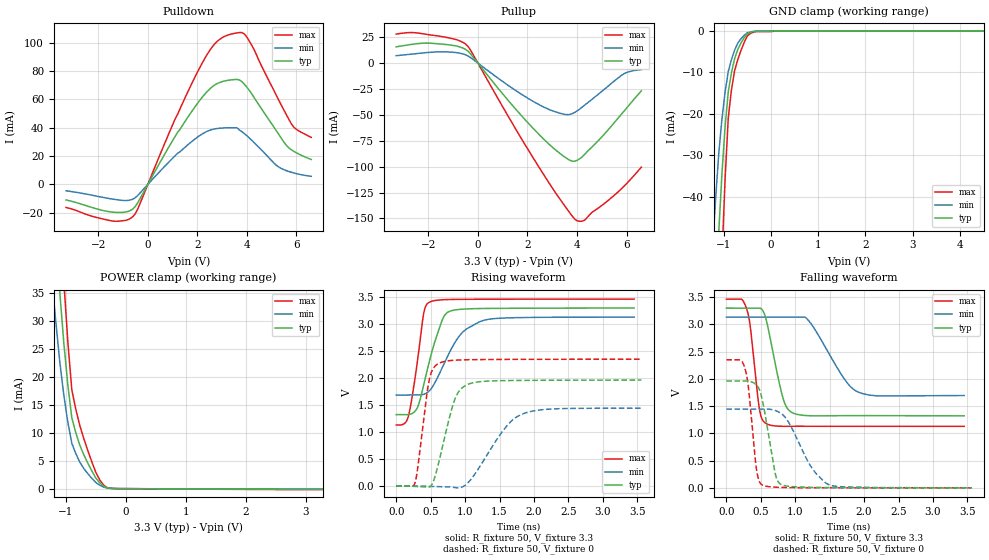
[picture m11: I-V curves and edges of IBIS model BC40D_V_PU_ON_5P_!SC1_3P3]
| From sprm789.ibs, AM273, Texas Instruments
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|   Model Cell BC40D_V_PU_ON_5P_!SC1_3P3
|BC40D_V_PU_ON_5P_!SC1_3P3
[Model]   BC40D_V_PU_ON_5P_!SC1_3P3
Model_type   I/O
Polarity   Non-Inverting
Enable   Active-Low
Vinl =  0.8V
Vinh =  2V
Cref =  15pF
Rref =  100.0000M
Vref =  0V
Vmeas =  1.65
C_comp   2.059994p   1.862014p   2.067327p
|[Input load] weak_pu_on
|[Output drive] fast
|[supplytol] 5
|[temp] ind
[Model Spec]
Vinl   0.8V   0.8V   0.8V
Vinh   2V   2V   2V
[Temperature Range]   25   125   -40
[Voltage Range]   3.3   3.135   3.465
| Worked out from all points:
|   slope of the pulldown table from 0 to 0.495 V, typ, clamps not added: 31.8 ohm
|   slope of the pullup table from 0 to 0.495 V, typ, clamps not added: 33.3 ohm
|   GND clamp passes 1 mA (typ) near -0.52 V on its own axis
|   POWER clamp passes 1 mA (typ) near -0.43 V on its own axis
|   rising waveform, R_fixture 50, V_fixture 3.3: 20-80 % time 251ps typ, 370ps min, 151ps max; typ from 1.32 V to 3.3 V
|   rising waveform, R_fixture 50, V_fixture 0: 20-80 % time 232ps typ, 457ps min, 141ps max; typ from 0 V to 1.97 V
|   falling waveform, R_fixture 50, V_fixture 3.3: 20-80 % time 196ps typ, 407ps min, 120ps max; typ from 3.3 V to 1.32 V
|   falling waveform, R_fixture 50, V_fixture 0: 20-80 % time 159ps typ, 360ps min, 107ps max; typ from 1.96 V to 0.002 V
| Nom Voltages:
|   VDD=1.1, VDDS=3.3, VDDS18=1.8, ESD_BIASFET=0, VSS=0, VSSS=0
| Min Voltages:
|   VDD=1.045, VDDS=3.135, VDDS18=1.71, ESD_BIASFET=0, VSS=0, VSSS=0
| Max Voltages:
|   VDD=1.16, VDDS=3.465, VDDS18=1.89, ESD_BIASFET=0, VSS=0, VSSS=0
[POWER_clamp]
|   voltage   I(typ)   I(min)   I(max)
-3.3V     446.9mA    437.1mA    604mA
-1.233V   56.55mA    37.5mA     80.28mA
-1.167V   45.63mA    29.89mA    65.07mA
-1.1V     35.1mA     22.65mA    50.26mA
-1.033V   26.08mA    16.75mA    37.2mA
-966.7mV  18.62mA    11.92mA    26.34mA
-900mV    12.7mA     8.144mA    17.7mA
-833.3mV  10mA       6.261mA    14.22mA
-766.7mV  7.795mA    4.75mA     11.31mA
-566.7mV  3.199mA    1.871mA    4.824mA
-366.7mV  433.5uA    268.9uA    617.1uA
3.3V      -100.3uA   -54.66uA   -173.1uA
[Pulldown]
|   voltage   I(typ)   I(min)   I(max)
-3.3V     -10.92mA   -4.469mA   -16.24mA
-1.4V     -19.52mA   -10.37mA   -25.81mA
-600mV    -17.22mA   -10.34mA   -22.6mA
-400mV    -12.67mA   -7.623mA   -17.05mA
1.2V      36.7mA     21.92mA    49.35mA
2.1V      59.3mA     34.49mA    82.4mA
2.7V      70.09mA    39.15mA    99.03mA
3.3V      73.56mA    39.95mA    105.7mA
3.9V      70.66mA    35.84mA    106mA
5.2V      37.64mA    13.39mA    62.46mA
5.8V      24.43mA    8.578mA    42.66mA
6.6V      17.6mA     5.765mA    33.17mA
[Pullup]
|   voltage   I(typ)   I(min)   I(max)
-3.3V     15.77mA    7.22mA     28.03mA
-2.7V     18.05mA    8.673mA    29.54mA
-1.9V     19.23mA    10.53mA    27.2mA
-900mV    16.69mA    10.25mA    22.94mA
-400mV    11.53mA    6.969mA    16.15mA
1.4V      -40.96mA   -24.37mA   -58.54mA
2.6V      -72.01mA   -41.71mA   -105.6mA
3.6V      -92.16mA   -49.74mA   -141mA
4V        -93.89mA   -46.2mA    -152.2mA
4.3V      -88.33mA   -40.72mA   -151.7mA
5.9V      -46.29mA   -10.2mA    -118.8mA
6.6V      -26.71mA   -6.269mA   -100.4mA
[GND_clamp]
|   voltage   I(typ)   I(min)   I(max)
-3.3V     -787.2mA   -627.7mA   -1.235A
-1.233V   -85.67mA   -52.14mA   -138.8mA
-1.167V   -66.48mA   -40.37mA   -107.8mA
-1.1V     -48.26mA   -29.38mA   -78.01mA
-1.033V   -34.3mA    -21.2mA    -54.61mA
-966.7mV  -23.1mA    -14.68mA   -35.59mA
-900mV    -14.66mA   -9.807mA   -20.94mA
-833.3mV  -10.12mA   -6.96mA    -14.29mA
-700mV    -4.501mA   -2.971mA   -6.963mA
-500mV    -717.7uA   -493.4uA   -1.261mA
100mV     0A         0A         0A
6.6V      0A         0A         0A
[Ramp]
| variable   typ   min   max
dV/dt_f  1.1950495/0.19765753n 0.88964479/0.4200289n  1.4061684/0.12033881n
dV/dt_r  1.1911245/0.23430808n 0.88879161/0.46777455n  1.4196341/0.14133941n
R_load = 50
[Rising Waveform]
R_fixture = 50
V_fixture = 3.3
V_fixture_min = 3.135
V_fixture_max = 3.465
|   time   V(typ)   V(min)   V(max)
0s        1.324V     1.688V     1.132V
178.2ps   1.325V     1.688V     1.3V
302ps     1.441V     1.688V     2.255V
397.2ps   1.866V     1.701V     3.188V
481.7ps   2.312V     1.767V     3.408V
652.6ps   3.023V     2.153V     3.452V
724.3ps   3.197V     2.349V     3.456V
949.9ps   3.277V     2.833V     3.461V
1.235ns   3.291V     3.056V     3.463V
3.453ns   3.299V     3.131V     3.465V
[Rising Waveform]
R_fixture = 50
V_fixture = 0
V_fixture_min = 0
V_fixture_max = 0
|   time   V(typ)   V(min)   V(max)
0s        0V         0V         2.107mV
272.8ps   -4.726mV   0V         61.13mV
474.5ps   -18.41mV   -3.512mV   1.937V
535.3ps   75.37mV    -5.14mV    2.176V
616.3ps   432.5mV    -7.541mV   2.273V
848.1ps   1.598V     -25.65mV   2.334V
1.041ns   1.886V     60.45mV    2.342V
1.574ns   1.955V     1.066V     2.348V
1.816ns   1.959V     1.327V     2.349V
3.559ns   1.965V     1.444V     2.352V
[Falling Waveform]
R_fixture = 50
V_fixture = 3.3
V_fixture_min = 3.135
V_fixture_max = 3.465
|   time   V(typ)   V(min)   V(max)
0s        3.299V     3.134V     3.464V
297.1ps   3.299V     3.134V     3.277V
347.5ps   3.299V     3.134V     2.96V
479.3ps   3.299V     3.134V     1.457V
583.2ps   3.064V     3.134V     1.178V
818.9ps   1.664V     3.134V     1.132V
962ps     1.378V     3.134V     1.132V
1.185ns   1.327V     3.084V     1.132V
1.91ns    1.327V     1.762V     1.131V
3.453ns   1.324V     1.696V     1.131V
[Falling Waveform]
R_fixture = 50
V_fixture = 0
V_fixture_min = 0
V_fixture_max = 0
|   time   V(typ)   V(min)   V(max)
0s        1.964V     1.449V     2.351V
273.4ps   1.964V     1.449V     2.18V
323.9ps   1.96V      1.449V     1.807V
434.9ps   1.893V     1.449V     362.2mV
522.6ps   1.613V     1.449V     54.33mV
709.6ps   264mV      1.421V     15.11mV
807.1ps   57.02mV    1.356V     10.14mV
1.237ns   12.08mV    376.7mV    4.232mV
1.49ns    8.452mV    59.61mV    3.21mV
3.559ns   2.489mV    4.507mV    2.796mV
